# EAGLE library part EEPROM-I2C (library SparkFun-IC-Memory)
I2C EEPROMs, 24LC256 and others 24LC256 Series 256 kb I2C 2 Wire (32 k x 8 Bit) 2.5 V Serial EEPROM SMD - SOIC-8 Datasheet SparkFun Products SparkFun UDB5 - PIC UAV Development Board (GPS-11703)
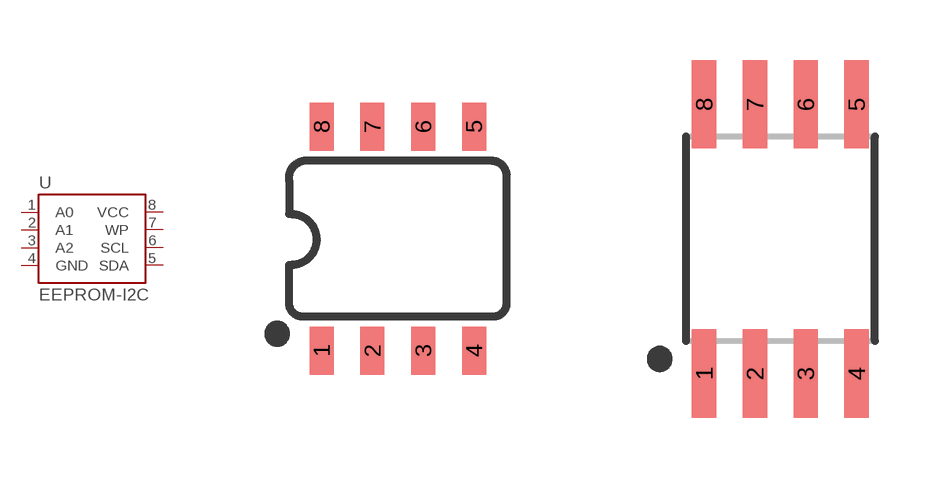
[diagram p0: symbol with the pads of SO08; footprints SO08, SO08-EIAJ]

Designator prefix U

## EEPROM-I2C256K (PROD_ID: IC-09714; VALUE: 24LC256)  [SO08]
1  A0
2  A1
3  A2
4  GND  pwr
5  SDA
6  SCL
7  WP
8  VCC  pwr

## EEPROM-I2CEIAJ (PROD_ID: NA-XXXXX; VALUE: I2C EEPROM)  [SO08-EIAJ]
Pads as for SO08

## EEPROM-I2C512K (PROD_ID: IC-14645)  [SO08]
Pads as for SO08

## Footprint SO08 (pad centres in mm)
SOIC, 0.15 inch width
smd 0.6 x 1.2: 1 -1.905,-2.8; 2 -0.635,-2.8; 3 0.635,-2.8; 4 1.905,-2.8; 5 1.905,2.8; 6 0.635,2.8; 7 -0.635,2.8; 8 -1.905,2.8

## Footprint SO08-EIAJ (pad centres in mm)
Fits EIAJ packages (wide version of the SOIC-8).
smd 0.61 x 2.21: 1 -1.905,-3.378; 2 -0.635,-3.378; 3 0.635,-3.378; 4 1.905,-3.378; 5 1.905,3.353; 6 0.635,3.353; 7 -0.635,3.353; 8 -1.905,3.353

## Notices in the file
Licensing: Creative Commons ShareAlike 4.0 International - https://creativecommons.org/licenses/by-sa/4.0
